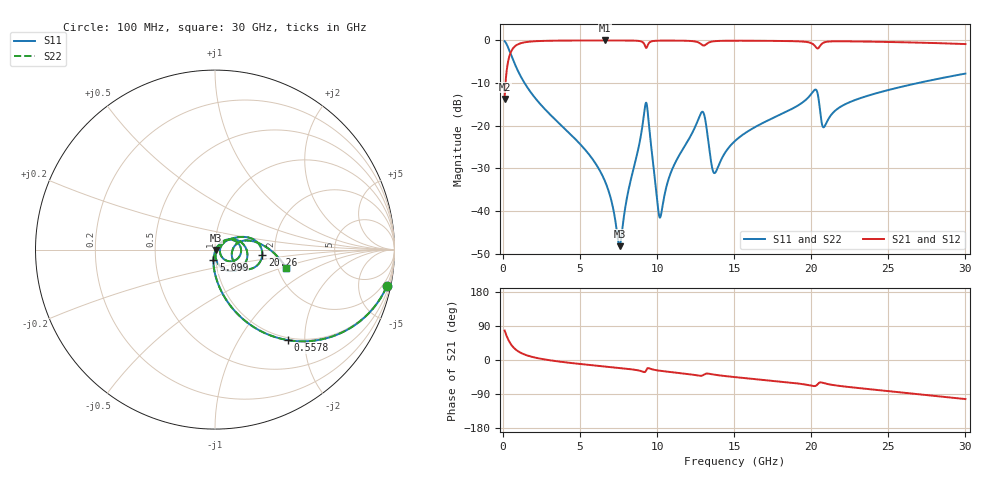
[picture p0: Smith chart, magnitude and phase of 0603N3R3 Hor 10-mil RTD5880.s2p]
# GHz S MA R 50
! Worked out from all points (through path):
!   3201 points, 100 MHz to 30 GHz, reference 50 ohm
!   highest |S21| = -0.03 dB at 6.585 GHz (marker M1); lowest = -13.8 dB at 100 MHz (marker M2)
!   group delay of S21, straight-line fit = 10.9 ps
!   lowest |S11| = -48.2 dB at 7.556 GHz (marker M3), VSWR 1.01, Z = 50.4 - j0.156 ohm
!   |S11| at or under -10 dB: 1.393 GHz to 26.93 GHz (25.54 GHz wide, 180 % of centre)
!   |S22| runs from -48.2 to -0.2 dB; largest |S21 - S12| = 0
!   S11 on the Smith chart (normalised r, x): 100 MHz: 0.96, -9.32; 557.8 MHz: 0.96, -1.66; 5.099 GHz: 0.98, -0.11; 20.26 GHz: 1.71, -0.11; 30 GHz: 2.22, -0.54
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0.1  0.9787 -12.1  0.2051 77.9  0.2051 77.9  0.9787 -12.1
0.5578437  0.6481 -51.1  0.7609 38.8  0.7609 38.8  0.6481 -51.1
1.632375  0.2711 -78.6  0.9612 11.1  0.9612 11.1  0.2711 -78.6
5.089563  0.05837 -98.4  0.9957 -10.9  0.9957 -10.9  0.05837 -98.4
5.098906  0.05812 -98.4  0.9957 -10.9  0.9957 -10.9  0.05812 -98.4
6.584562  0.02295 -99.3  0.9965 -17.1  0.9965 -17.1  0.02295 -99.3
7.556312  0.00387 -23.7  0.996 -21.1  0.996 -21.1  0.00387 -23.7
9.256875  0.1833 -9.0  0.8261 -29.4  0.8261 -29.4  0.1833 -9.0
9.415719  0.1277 -62.5  0.9002 -21.4  0.9002 -21.4  0.1277 -62.5
10.06978  0.01024 -53.0  0.9906 -27.7  0.9906 -27.7  0.01024 -53.0
10.23797  0.008851 -1.1  0.992 -28.7  0.992 -28.7  0.008851 -1.1
10.95744  0.03029 45.6  0.993 -32.1  0.993 -32.1  0.03029 45.6
12.87291  0.1431 5.2  0.8963 -41.6  0.8963 -41.6  0.1431 5.2
13.09716  0.1237 -30.0  0.8769 -37.1  0.8769 -37.1  0.1237 -30.0
13.7045  0.0278 -7.2  0.976 -38.6  0.976 -38.6  0.0278 -7.2
15.05  0.06617 37.9  0.9896 -45.2  0.9896 -45.2  0.06617 37.9
20.03956  0.2405 9.5  0.9199 -68.0  0.9199 -68.0  0.2405 9.5
20.26381  0.2649 -6.5  0.8476 -68.5  0.8476 -68.5  0.2649 -6.5
20.83378  0.09656 -3.4  0.9448 -61.1  0.9448 -61.1  0.09656 -3.4
22.03912  0.1722 17.0  0.9741 -69.4  0.9741 -69.4  0.1722 17.0
25.01978  0.2621 6.1  0.9569 -82.2  0.9569 -82.2  0.2621 6.1
30  0.4077 -14.3  0.9042 -103.1  0.9042 -103.1  0.4077 -14.3
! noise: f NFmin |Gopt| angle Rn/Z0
0.1  0.0003864  0.9391  0.8334  0.001416
3.417  0.003912  0.8046  9.739  0.004129
6.743  0.006874  0.784  18.87  0.006363
10.06  0.01429  0.8411  27.97  0.01796
13.39  0.03929  0.9206  36.97  0.09843
16.7  0.01558  0.772  45.56  0.01188
20.03  0.04747  0.9048  54.33  0.0866
23.35  0.02028  0.7628  62.34  0.01279
26.67  0.0215  0.7499  70.25  0.01171
30  0.02399  0.7514  77.99  0.01191
